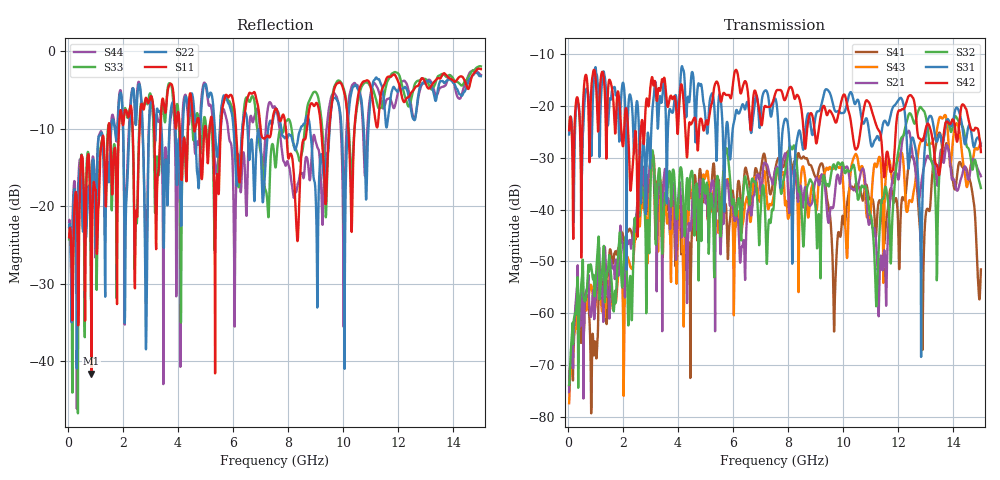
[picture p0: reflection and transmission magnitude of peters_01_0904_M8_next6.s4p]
# MHZ S RI R 50.00
! FREQ  S11  S12  S13  S14
!  S21  S22  S23  S24
!  S31  S32  S33  S34
!  S41  S42  S43  S44
!  REAL  IMAG  REAL  IMAG  REAL  IMAG  REAL  IMAG
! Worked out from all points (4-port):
!   1496 points, 50 MHz to 15 GHz, reference 50 ohm
!   strongest paths, dB at 50 MHz, 3.79 GHz, 7.53 GHz, 11.27 GHz, 15 GHz:
!     S42: -24.7, -18.6, -17.7, -24.6, -28.9
!     S31: -25.5, -21.3, -18.6, -26.0, -27.7
!     S32: -73.8, -33.9, -35.0, -49.8, -35.9
!     S21: -75.1, -35.3, -32.4, -56.5, -33.6
!     S43: -77.3, -40.8, -35.3, -30.5, -27.3
!     S41: -74.0, -37.4, -32.3, -39.1, -51.5
!   lowest |S11| = -41.6 dB at 860 MHz (marker M1), VSWR 1.02, Z = 50.6 + j0.602 ohm
!   |S11| at or under -10 dB: start of sweep to 1.472 GHz; 7.003 GHz to 7.4 GHz (396.8 MHz wide, 5.51 % of centre); 7.921 GHz to 8.682 GHz (761.2 MHz wide, 9.17 % of centre)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
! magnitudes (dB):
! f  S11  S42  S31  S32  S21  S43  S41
! 50 MHz  -24.0  -24.7  -25.5  -73.8  -75.1  -77.3  -74.0
! 860 MHz  -41.6  -16.3  -29.7  -51.2  -60.2  -54.7  -77.8
! 3.04 GHz  -5.8  -14.8  -23.9  -30.3  -30.4  -30.6  -29.8
! 9.69 GHz  -4.7  -22.8  -20.9  -31.6  -37.5  -31.9  -59.0
! 12.88 GHz  -3.5  -26.8  -38.0  -20.7  -33.3  -26.5  -67.0
! 13.49 GHz  -3.5  -33.2  -25.5  -33.4  -31.3  -22.4  -25.2
! 15 GHz  -2.3  -28.9  -27.7  -35.9  -33.6  -27.3  -51.5
